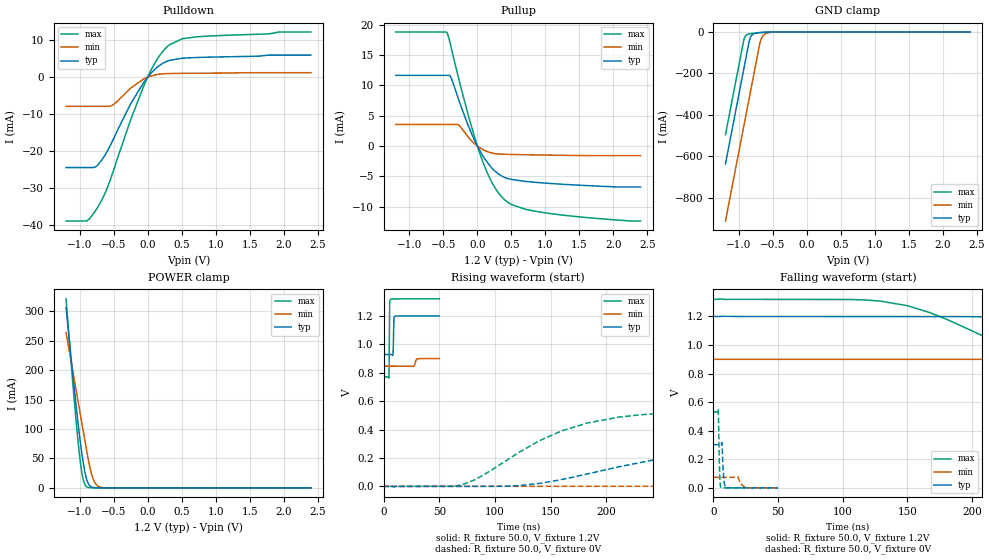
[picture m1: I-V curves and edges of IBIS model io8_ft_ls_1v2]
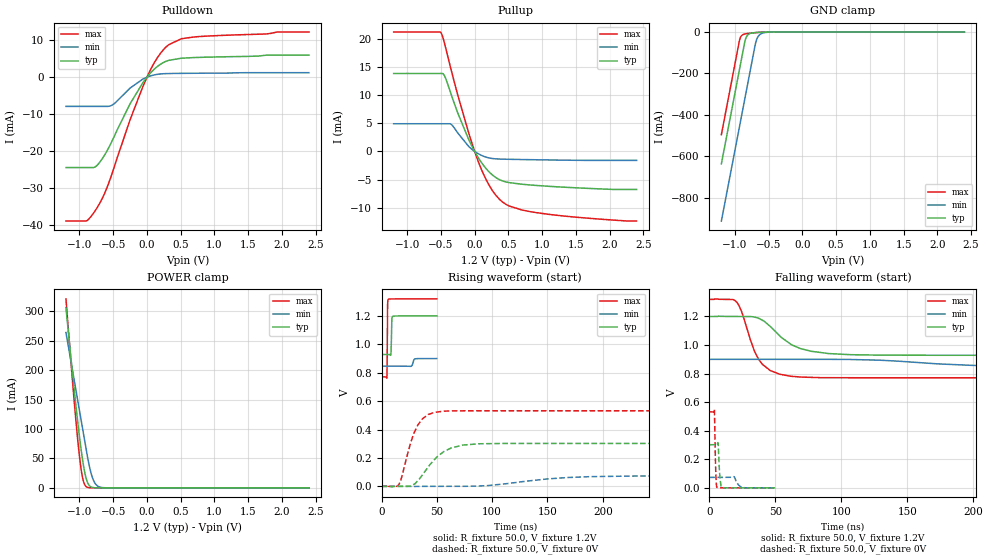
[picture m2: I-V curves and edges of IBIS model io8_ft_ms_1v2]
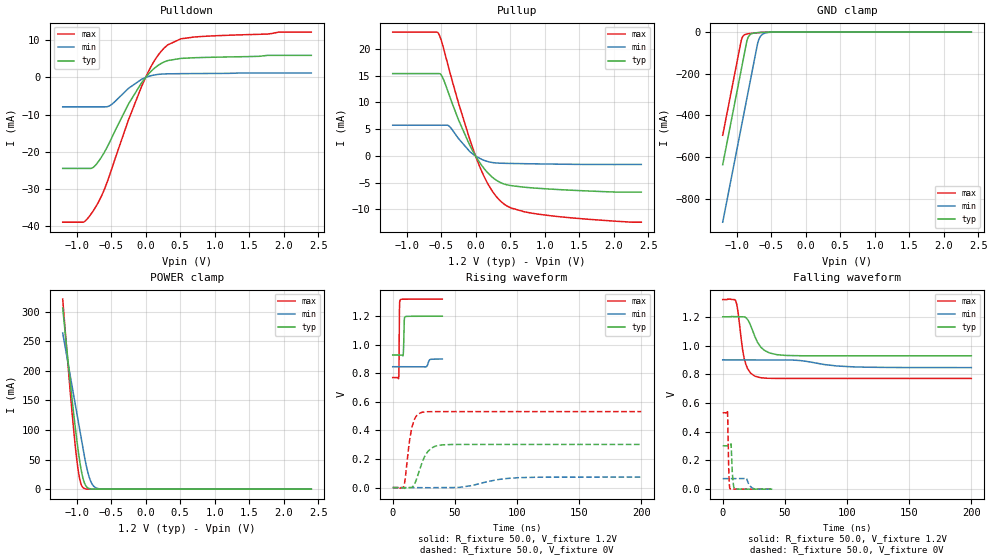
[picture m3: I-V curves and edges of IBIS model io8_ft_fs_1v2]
|   IBIS file stm32l452_lqfp64_p.ibs
[IBIS ver] 4.2
[File name] stm32l452_lqfp64_p.ibs
[File Rev] 3.0
[Date]  05-04-2021
[Source] Data Created at STMicroelectronics
[Disclaimer]  This information is for modeling purpose only and is
   not guaranted. The information is subject to change without
   notice.
[Copyright] Copyright 2021 STMicroelectronics Inc.
|   Component stm32l452_lqfp64_p
[Component] stm32l452_lqfp64_p
[Manufacturer] STMicroelectronics
[Package]
| variable   typ   min   max
R_pkg   0.0   0.0   0.0
L_pkg   0.0H   0.0H   0.0H
C_pkg   0.0F   0.0F   0.0F
[Pin]  signal_name   model_name   R_pin   L_pin   C_pin
1 VBAT POWER 68.980E-3 4.220E-9 120.000E-15
2 PC13 io8_ft 63.756E-3 3.679E-9 93.469E-15
3 PC14-OSC32_IN io8_ft 59.336E-3 3.221E-9 71.020E-15
4 PC15-OSC32_OUT io8_ft 55.719E-3 2.846E-9 52.653E-15
5 PH0-OSC_IN io8_ft 52.907E-3 2.555E-9 38.367E-15
6 PH1-OSC_OUT io8_ft 50.897E-3 2.347E-9 28.163E-15
7 NRST ioreset_ft_v33 49.692E-3 2.222E-9 22.041E-15
8 PC0 io8_ft_i2c 49.290E-3 2.180E-9 20.000E-15
9 PC1 io8_ft_i2c 49.290E-3 2.180E-9 20.000E-15
10 PC2 io8_ft 49.692E-3 2.222E-9 22.041E-15
11 PC3 io8_ft 50.897E-3 2.347E-9 28.163E-15
12 VSSA/VREF- GND 52.907E-3 2.555E-9 38.367E-15
13 VDDA/VREF+ POWER 55.719E-3 2.846E-9 52.653E-15
14 PA0 io8_ft 59.336E-3 3.221E-9 71.020E-15
15 PA1 io8_ft 63.756E-3 3.679E-9 93.469E-15
16 PA2 io8_ft 68.980E-3 4.220E-9 120.000E-15
17 PA3 io8_ft 68.980E-3 4.220E-9 120.000E-15
18 VSS GND 63.756E-3 3.679E-9 93.469E-15
19 VDD POWER 59.336E-3 3.221E-9 71.020E-15
20 PA4 io8_ft 55.719E-3 2.846E-9 52.653E-15
21 PA5 io8_ft 52.907E-3 2.555E-9 38.367E-15
22 PA6 io8_ft 50.897E-3 2.347E-9 28.163E-15
23 PA7 io8_ft_i2c 49.692E-3 2.222E-9 22.041E-15
24 PC4 io8_ft 49.290E-3 2.180E-9 20.000E-15
25 PB0 io8_ft 49.290E-3 2.180E-9 20.000E-15
26 PB1 io8_ft 49.692E-3 2.222E-9 22.041E-15
27 PB2 io8_ft 50.897E-3 2.347E-9 28.163E-15
28 PB10 io8_ft_i2c 52.907E-3 2.555E-9 38.367E-15
29 PB11 io8_ft_i2c 55.719E-3 2.846E-9 52.653E-15
30 VDD12 POWER 59.336E-3 3.221E-9 71.020E-15
31 VSS GND 63.756E-3 3.679E-9 93.469E-15
32 VDD POWER 68.980E-3 4.220E-9 120.000E-15
33 PB12 io8_ft 68.980E-3 4.220E-9 120.000E-15
34 PB13 io8_ft_i2c 63.756E-3 3.679E-9 93.469E-15
35 PB14 io8_ft_i2c 59.336E-3 3.221E-9 71.020E-15
36 PB15 io8_ft 55.719E-3 2.846E-9 52.653E-15
37 PC6 io8_ft 52.907E-3 2.555E-9 38.367E-15
38 PC7 io8_ft 50.897E-3 2.347E-9 28.163E-15
39 PC8 io8_ft 49.692E-3 2.222E-9 22.041E-15
40 PC9 io8_ft 49.290E-3 2.180E-9 20.000E-15
41 PA8 io8_ft 49.290E-3 2.180E-9 20.000E-15
42 PA9 io8_ft_i2c 49.692E-3 2.222E-9 22.041E-15
43 PA10 io8_ft_i2c 50.897E-3 2.347E-9 28.163E-15
44 PA11 io8_usb_lsfs_bcd_otg20_ft 52.907E-3 2.555E-9 38.367E-15
45 PA12 io8_usb_lsfs_bcd_otg20_ft 55.719E-3 2.846E-9 52.653E-15
46 PA13 io8_ft 59.336E-3 3.221E-9 71.020E-15
47 VSS GND 63.756E-3 3.679E-9 93.469E-15
48 VDDUSB POWER 68.980E-3 4.220E-9 120.000E-15
49 PA14 io8_ft 68.980E-3 4.220E-9 120.000E-15
50 PA15 io8_ft 63.756E-3 3.679E-9 93.469E-15
51 PC10 io8_ft 59.336E-3 3.221E-9 71.020E-15
52 PC11 io8_ft 55.719E-3 2.846E-9 52.653E-15
53 PC12 io8_ft 52.907E-3 2.555E-9 38.367E-15
54 PB3 io8_ft 50.897E-3 2.347E-9 28.163E-15
55 PB4 io8_ft_i2c 49.692E-3 2.222E-9 22.041E-15
56 PB5 io8_ft 49.290E-3 2.180E-9 20.000E-15
57 PB6 io8_ft_i2c 49.290E-3 2.180E-9 20.000E-15
58 PB7 io8_ft_i2c 49.692E-3 2.222E-9 22.041E-15
59 PH3-BOOT0 io8_ft 50.897E-3 2.347E-9 28.163E-15
60 PB8 io8_ft_i2c 52.907E-3 2.555E-9 38.367E-15
61 PB9 io8_ft_i2c 55.719E-3 2.846E-9 52.653E-15
62 VDD12 POWER 59.336E-3 3.221E-9 71.020E-15
63 VSS GND 63.756E-3 3.679E-9 93.469E-15
64 VDD POWER 68.980E-3 4.220E-9 120.000E-15
[Model Selector] io8_ft
io8_ft_ls_1v2   "GPIO - 5V tolerant - 1.2V range - Low speed"
io8_ft_ms_1v2   "GPIO - 5V tolerant - 1.2V range - Med speed"
io8_ft_fs_1v2   "GPIO - 5V tolerant - 1.2V range - Fast speed"
io8_ft_hs_1v2   "GPIO - 5V tolerant - 1.2V range - High speed"
io8_ft_ls_1v8   "GPIO - 5V tolerant - 1.8V range - Low speed"
io8_ft_ms_1v8   "GPIO - 5V tolerant - 1.8V range - Med speed"
io8_ft_fs_1v8   "GPIO - 5V tolerant - 1.8V range - Fast speed"
io8_ft_hs_1v8   "GPIO - 5V tolerant - 1.8V range - High speed"
io8_ft_ls_3v3   "GPIO - 5V tolerant - 3.3V range - Low speed"
io8_ft_ms_3v3   "GPIO - 5V tolerant - 3.3V range - Med speed"
io8_ft_fs_3v3   "GPIO - 5V tolerant - 3.3V range - Fast speed"
io8_ft_hs_3v3   "GPIO - 5V tolerant - 3.3V range - High speed"
[Model Selector] io8_ft_i2c
io8_ft_ls_1v2   "GPIO - 5V tolerant - 1.2V range - Low speed"
io8_ft_ms_1v2   "GPIO - 5V tolerant - 1.2V range - Med speed"
io8_ft_fs_1v2   "GPIO - 5V tolerant - 1.2V range - Fast speed"
io8_ft_hs_1v2   "GPIO - 5V tolerant - 1.2V range - High speed"
io8_ft_ls_1v8   "GPIO - 5V tolerant - 1.8V range - Low speed"
io8_ft_ms_1v8   "GPIO - 5V tolerant - 1.8V range - Med speed"
io8_ft_fs_1v8   "GPIO - 5V tolerant - 1.8V range - Fast speed"
io8_ft_hs_1v8   "GPIO - 5V tolerant - 1.8V range - High speed"
io8_ft_ls_3v3   "GPIO - 5V tolerant - 3.3V range - Low speed"
io8_ft_ms_3v3   "GPIO - 5V tolerant - 3.3V range - Med speed"
io8_ft_fs_3v3   "GPIO - 5V tolerant - 3.3V range - Fast speed"
io8_ft_hs_3v3   "GPIO - 5V tolerant - 3.3V range - High speed"
io8_ft_i2c_1v2   "GPIO - 5V tolerant - 1.2V range - Open drain"
io8_ft_i2c_1v8   "GPIO - 5V tolerant - 1.8V range - Open drain"
io8_ft_i2c_3v3   "GPIO - 5V tolerant - 3.3V range - Open drain"
[Model Selector] io8_usb_lsfs_bcd_otg20_ft
io8_ft_ls_1v2   "GPIO - 5V tolerant - 1.2V range - Low speed"
io8_ft_ms_1v2   "GPIO - 5V tolerant - 1.2V range - Med speed"
io8_ft_fs_1v2   "GPIO - 5V tolerant - 1.2V range - Fast speed"
io8_ft_hs_1v2   "GPIO - 5V tolerant - 1.2V range - High speed"
io8_ft_ls_1v8   "GPIO - 5V tolerant - 1.8V range - Low speed"
io8_ft_ms_1v8   "GPIO - 5V tolerant - 1.8V range - Med speed"
io8_ft_fs_1v8   "GPIO - 5V tolerant - 1.8V range - Fast speed"
io8_ft_hs_1v8   "GPIO - 5V tolerant - 1.8V range - High speed"
io8_ft_ls_3v3   "GPIO - 5V tolerant - 3.3V range - Low speed"
io8_ft_ms_3v3   "GPIO - 5V tolerant - 3.3V range - Med speed"
io8_ft_fs_3v3   "GPIO - 5V tolerant - 3.3V range - Fast speed"
io8_ft_hs_3v3   "GPIO - 5V tolerant - 3.3V range - High speed"
io8usb_ft_hs_3v3   "USB full speed"
io8usb_ft_ls_3v3   "USB low speed"
|[Model Selector] ioreset_ft_v33
|ioreset_ft_v33_1v2   "Reset PAD. 5V tolerant. 1.2V range"
|ioreset_ft_v33_1v8   "Reset PAD. 5V tolerant. 1.8V range"
|ioreset_ft_v33_3v3   "Reset PAD. 5V tolerant. 3.3V range"
[Model Selector] ioreset_ft_v33
ioreset_1v2_pu  "RESET 1.2V range with PU"
ioreset_1v2  "RESET 1.2V range"
ioreset_1v8_pu  "RESET 1.8V range with PU"
ioreset_1v8  "RESET 1.8V range"
ioreset_3v3_pu  "RESET 3.3V range with PU"
ioreset_3v3  "RESET 3.3V range"
| Models and submodels in the file (23): io8_ft_ls_1v2 (I/O), io8_ft_ms_1v2 (I/O), io8_ft_fs_1v2 (I/O), io8_ft_hs_1v2 (I/O), io8_ft_ls_1v8 (I/O), io8_ft_ms_1v8 (I/O), io8_ft_fs_1v8 (I/O), io8_ft_hs_1v8 (I/O), io8_ft_ls_3v3 (I/O), io8_ft_ms_3v3 (I/O), io8_ft_fs_3v3 (I/O), io8_ft_hs_3v3 (I/O), io8_ft_i2c_1v2 (I/O_open_drain), io8_ft_i2c_1v8 (I/O_open_drain), io8_ft_i2c_3v3 (I/O_open_drain), io8usb_ft_hs_3v3 (I/O), io8usb_ft_ls_3v3 (I/O), ioreset_1v2_pu (I/O_open_drain), ioreset_1v2 (I/O_open_drain), ioreset_1v8_pu (I/O_open_drain), ioreset_1v8 (I/O_open_drain), ioreset_3v3_pu (I/O_open_drain), ioreset_3v3 (I/O_open_drain)
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[Model]   io8_ft_ls_1v2
Model_type I/O
Polarity   Non-Inverting
Enable   Active-Low
| CAP_THRESHOLD on pad IOFT is "UDTCAPC" :
| Rising=30.00f vddiom   Falling=70.00f vddiom
| C_comp min and max val. don't necessarily correlate with the min and max pvt
| but are the smallest and greatest pad capacitance found.
| var   typ   min   max
C_comp   1.83455pF  1.76050pF  1.83491pF
|C_comp_pullup   1.06365pF  1.01770pF  1.04720pF
|C_comp_pulldown   770.90000fF  742.80001fF  787.71000fF
Vinl = 270.0mV
Vinh = 924.0mV
Vmeas = 600.0mV   | Reference voltage for timing measurements
Cref  = 50.0pF   | Timing specification test load capacitance value
Rref  = 100.0MOhm   | Timing specification test load resistance value
Vref  = 600.0mV   | Timing specification test load voltage
[Model Spec]
| TIME_THRESHOLD on pin ZIV12 is "CMOS" :
| Rising=50.00f vdd   Falling=50.00f vdd
Vinl 458.70000mV 364.70000mV 499.70000mV
Vinh 728.30000mV 548.30000mV 792.30000mV
| variable   typ   min   max
[Temperature Range] 25.0 140.0 -40.0
| variable   typ   min   max
[Voltage Range] 1.2V 900.0mV 1.32V
| variable   typ   min   max
[POWER Clamp Reference] 1.2V 900.0mV 1.32V
| variable   typ   min   max
[GND Clamp Reference] 0V 0V 0V
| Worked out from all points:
|   slope of the pulldown table from 0 to 0.18 V, typ, clamps not added: 55.6 ohm
|   slope of the pullup table from 0 to 0.18 V, typ, clamps not added: 56.3 ohm
|   GND clamp passes 1 mA (typ) near -0.61 V on its own axis
|   POWER clamp passes 1 mA (typ) near -0.81 V on its own axis
|   rising waveform, R_fixture 50.0, V_fixture 1.2V: 20-80 % time 432ps typ, 1.3ns min, 278ps max; typ from 0.928 V to 1.2 V
|   falling waveform, R_fixture 50.0, V_fixture 1.2V: 20-80 % time 167ns typ, 491ns min, 99.5ns max; typ from 1.2 V to 0.928 V
|   rising waveform, R_fixture 50.0, V_fixture 0V: 20-80 % time 127ns typ, 295ns min, 78.9ns max; typ from 0 V to 0.302 V
|   falling waveform, R_fixture 50.0, V_fixture 0V: 20-80 % time 1.14ns typ, 2.98ns min, 786ps max; typ from 0.302 V to 0 V
[POWER Clamp]
-1.2V     306.2mA    263.9mA    321.2mA
-1.09V    180mA      191mA      163.4mA
-1.05V    136.9mA    164.5mA    110.9mA
-1.01V    96.55mA    138mA      64.02mA
-960mV    52.29mA    104.9mA    20.68mA
-930mV    31.08mA    85.01mA    7.282mA
-900mV    15.67mA    65.13mA    2.025mA
-850mV    3.417mA    35.2mA     196.2uA
-800mV    570.2uA    14.97mA    18.13uA
-750mV    88.98uA    4.952mA    1.667uA
-680mV    6.495uA    823.9uA    58.96nA
2.4V      0A         0A         0A
[GND Clamp]
-1.2V     -636.9mA   -913.2mA   -495.8mA
-940mV    -194.9mA   -471.2mA   -53.78mA
-920mV    -160.9mA   -437.2mA   -28.06mA
-890mV    -109.9mA   -386.2mA   -14.28mA
-850mV    -43.09mA   -318.2mA   -9.18mA
-820mV    -18.33mA   -267.2mA   -7.516mA
-780mV    -7.695mA   -199.2mA   -5.87mA
-690mV    -2.548mA   -49.42mA   -2.9mA
-660mV    -1.868mA   -24.06mA   -2.112mA
-630mV    -1.326mA   -12.18mA   -1.447mA
-430mV    -19.32uA   -177.8uA   -8.091uA
2.4V      300pA      77.2nA     208.1pA
| variable   typ   min   max
[Pullup Reference] 1.2V 900.0mV 1.32V
| variable   typ   min   max
[Pulldown Reference] 0V 0V 0V
[Pullup]
-1.2V     11.66mA    3.558mA    18.8mA
-450mV    11.66mA    3.558mA    18.75mA
-390mV    11.34mA    3.558mA    16.48mA
-280mV    7.814mA    3.503mA    11.36mA
-110mV    2.689mA    1.153mA    4.138mA
50mV      -1.039mA   -379.5uA   -1.685mA
140mV     -2.617mA   -893.8uA   -4.276mA
240mV     -3.942mA   -1.22mA    -6.527mA
430mV     -5.313mA   -1.379mA   -9.149mA
700mV     -5.836mA   -1.444mA   -10.42mA
1.08V     -6.193mA   -1.513mA   -11.17mA
2.4V      -6.768mA   -1.592mA   -12.38mA
[Pulldown]
-1.2V     -24.47mA   -7.9mA     -38.94mA
-890mV    -24.47mA   -7.9mA     -38.83mA
-720mV    -23.49mA   -7.9mA     -34.76mA
-610mV    -20.54mA   -7.9mA     -30.69mA
-510mV    -17.01mA   -7.489mA   -25.69mA
-250mV    -7.205mA   -2.955mA   -11.53mA
0V        -16fA      0A         0A
160mV     2.97mA     779.8uA    5.417mA
320mV     4.547mA    983.4uA    8.763mA
510mV     5.135mA    1.031mA    10.4mA
700mV     5.311mA    1.057mA    10.88mA
2.4V      5.965mA    1.209mA    12.22mA
[Ramp]
dV/dt_r 181.26172mV/127.09367ns 44.06031mV/295.17618ns 319.20445mV/78.91734ns
dV/dt_f 162.93173mV/166.53891ns 32.17941mV/468.67509ns 329.57818mV/99.46975ns
R_load = 50.0
| Removed startup time: 0s 0s 0s  .
| Removed end time: 49.9ns.
[Rising Waveform]
R_fixture   = 50.0
V_fixture   = 1.2V
V_fixture_min = 900.0mV
V_fixture_max = 1.32V
0s        928.4mV    846.3mV    770.7mV
4.8ns     928.5mV    846.4mV    763.2mV
5.1ns     928.5mV    846.4mV    887.9mV
5.3ns     928.5mV    846.4mV    1.143V
5.5ns     928.5mV    846.4mV    1.284V
6.1ns     928.5mV    846.4mV    1.316V
8.4ns     926.5mV    846.4mV    1.32V
9.3ns     1.171V     846.4mV    1.32V
10.1ns    1.197V     846.4mV    1.32V
49.9ns    1.2V       899.9mV    1.32V
| Removed startup time: 0s 0s 0s  .
| Removed end time: 2.9999us.
[Falling Waveform]
R_fixture   = 50.0
V_fixture   = 1.2V
V_fixture_min = 900.0mV
V_fixture_max = 1.32V
0s        1.2V       900mV      1.32V
128.4ns   1.2V       900mV      1.309V
167.6ns   1.2V       900mV      1.227V
244ns     1.189V     900mV      938.9mV
267.2ns   1.176V     900mV      887.1mV
312.7ns   1.136V     900mV      829.5mV
416.9ns   1.017V     900mV      784.2mV
527.1ns   960.2mV    899.9mV    773.6mV
789.5ns   931.6mV    897.9mV    770.8mV
3us       928.4mV    846.4mV    770.7mV
| Removed startup time: 0s 0s 0s  .
| Removed end time: 1.9999us.
[Rising Waveform]
R_fixture   = 50.0
V_fixture   = 0V
V_fixture_min = 0V
V_fixture_max = 0V
0s        -21.55uV   -19.21uV   -16.72uV
70.8ns    -14.52uV   -5.362uV   12.13mV
121.2ns   5.11mV     -2.911uV   237.5mV
159.7ns   48.13mV    4.858uV    390.3mV
210.7ns   136.7mV    43.95uV    487mV
277.5ns   227.6mV    269.3uV    522.7mV
328.2ns   266.1mV    1.529mV    529.1mV
483.4ns   299.5mV    19.45mV    532mV
966.6ns   302.1mV    70.44mV    532mV
2us       302.1mV    73.43mV    532mV
| Removed startup time: 0s 0s 0s  .
| Removed end time: 49.9ns.
[Falling Waveform]
R_fixture   = 50.0
V_fixture   = 0V
V_fixture_min = 0V
V_fixture_max = 0V
0s        302.1mV    73.45mV    532mV
3.9ns     302.1mV    73.44mV    547.9mV
4.8ns     302mV      73.44mV    150.4mV
5.8ns     301.1mV    73.44mV    2.967mV
6.7ns     315mV      73.44mV    1.089mV
8.1ns     72.96mV    73.44mV    240.9uV
9.7ns     1.263mV    73.44mV    103.6uV
18.9ns    18.32uV    77.83mV    27.76uV
26.1ns    15.27uV    960.1uV    26.42uV
49.9ns    16.04uV    8.939uV    27.43uV
[Model]   io8_ft_ms_1v2
Model_type I/O
Polarity   Non-Inverting
Enable   Active-Low
| CAP_THRESHOLD on pad IOFT is "UDTCAPC" :
| Rising=30.00f vddiom   Falling=70.00f vddiom
| C_comp min and max val. don't necessarily correlate with the min and max pvt
| but are the smallest and greatest pad capacitance found.
| var   typ   min   max
C_comp   1.83454pF  1.76050pF  1.83490pF
|C_comp_pullup   1.06365pF  1.01770pF  1.04720pF
|C_comp_pulldown   770.89000fF  742.80001fF  787.70000fF
Vinl = 270.0mV
Vinh = 924.0mV
Vmeas = 600.0mV   | Reference voltage for timing measurements
Cref  = 50.0pF   | Timing specification test load capacitance value
Rref  = 100.0MOhm   | Timing specification test load resistance value
Vref  = 600.0mV   | Timing specification test load voltage
[Model Spec]
| TIME_THRESHOLD on pin ZIV12 is "CMOS" :
| Rising=50.00f vdd   Falling=50.00f vdd
Vinl 458.70000mV 364.70000mV 499.70000mV
Vinh 728.30000mV 548.30000mV 792.30000mV
| variable   typ   min   max
[Temperature Range] 25.0 140.0 -40.0
| variable   typ   min   max
[Voltage Range] 1.2V 900.0mV 1.32V
| variable   typ   min   max
[POWER Clamp Reference] 1.2V 900.0mV 1.32V
| variable   typ   min   max
[GND Clamp Reference] 0V 0V 0V
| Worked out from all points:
|   slope of the pulldown table from 0 to 0.18 V, typ, clamps not added: 55.6 ohm
|   slope of the pullup table from 0 to 0.18 V, typ, clamps not added: 56.3 ohm
|   GND clamp passes 1 mA (typ) near -0.61 V on its own axis
|   POWER clamp passes 1 mA (typ) near -0.81 V on its own axis
|   rising waveform, R_fixture 50.0, V_fixture 1.2V: 20-80 % time 434ps typ, 1.31ns min, 279ps max; typ from 0.928 V to 1.2 V
|   falling waveform, R_fixture 50.0, V_fixture 1.2V: 20-80 % time 22.8ns typ, 62.2ns min, 13.6ns max; typ from 1.2 V to 0.928 V
|   rising waveform, R_fixture 50.0, V_fixture 0V: 20-80 % time 20.6ns typ, 53.2ns min, 12.7ns max; typ from 0 V to 0.302 V
|   falling waveform, R_fixture 50.0, V_fixture 0V: 20-80 % time 1.14ns typ, 2.98ns min, 785ps max; typ from 0.302 V to 0 V
[POWER Clamp]
-1.2V     306.2mA    263.9mA    321.2mA
-1.09V    180mA      191mA      163.4mA
-1.05V    136.9mA    164.5mA    110.9mA
-1.01V    96.55mA    138mA      64.02mA
-960mV    52.29mA    104.9mA    20.68mA
-930mV    31.08mA    85.01mA    7.282mA
-900mV    15.67mA    65.13mA    2.025mA
-850mV    3.417mA    35.2mA     196.2uA
-800mV    570.2uA    14.97mA    18.13uA
-750mV    88.98uA    4.952mA    1.667uA
-680mV    6.495uA    823.9uA    58.96nA
2.4V      0A         0A         0A
[GND Clamp]
-1.2V     -636.9mA   -913.2mA   -495.8mA
-940mV    -194.9mA   -471.2mA   -53.78mA
-920mV    -160.9mA   -437.2mA   -28.06mA
-890mV    -109.9mA   -386.2mA   -14.28mA
-850mV    -43.09mA   -318.2mA   -9.18mA
-820mV    -18.33mA   -267.2mA   -7.516mA
-780mV    -7.695mA   -199.2mA   -5.87mA
-690mV    -2.548mA   -49.42mA   -2.9mA
-660mV    -1.868mA   -24.06mA   -2.112mA
-630mV    -1.326mA   -12.18mA   -1.447mA
-430mV    -19.32uA   -177.8uA   -8.091uA
2.4V      300pA      77.2nA     208.1pA
| variable   typ   min   max
[Pullup Reference] 1.2V 900.0mV 1.32V
| variable   typ   min   max
[Pulldown Reference] 0V 0V 0V
[Pullup]
-1.2V     13.87mA    4.927mA    21.25mA
-500mV    13.87mA    4.927mA    21.15mA
-450mV    13.53mA    4.927mA    19.38mA
-350mV    10.23mA    4.844mA    14.6mA
-90mV     2.161mA    908.5uA    3.352mA
40mV      -840.8uA   -309uA     -1.362mA
130mV     -2.46mA    -847.3uA   -4.016mA
230mV     -3.829mA   -1.199mA   -6.331mA
420mV     -5.274mA   -1.376mA   -9.06mA
510mV     -5.544mA   -1.401mA   -9.708mA
900mV     -6.043mA   -1.482mA   -10.87mA
2.4V      -6.768mA   -1.593mA   -12.38mA
[Pulldown]
-1.2V     -24.47mA   -7.9mA     -38.94mA
-890mV    -24.47mA   -7.9mA     -38.83mA
-720mV    -23.49mA   -7.9mA     -34.76mA
-610mV    -20.54mA   -7.9mA     -30.69mA
-510mV    -17.01mA   -7.49mA    -25.69mA
-250mV    -7.205mA   -2.955mA   -11.53mA
0V        -16fA      0A         0A
160mV     2.97mA     779.9uA    5.417mA
320mV     4.547mA    983.4uA    8.763mA
510mV     5.135mA    1.031mA    10.4mA
700mV     5.311mA    1.057mA    10.88mA
2.4V      5.965mA    1.209mA    12.22mA
[Ramp]
dV/dt_r 181.26477mV/20.56352ns 44.07195mV/53.14365ns 319.20364mV/12.72223ns
dV/dt_f 162.9258mV/22.80306ns 32.17064mV/62.22543ns 329.54886mV/13.59962ns
R_load = 50.0
| Removed startup time: 0s 0s 0s  .
| Removed end time: 49.9ns.
[Rising Waveform]
R_fixture   = 50.0
V_fixture   = 1.2V
V_fixture_min = 900.0mV
V_fixture_max = 1.32V
0s        928.4mV    846.3mV    770.7mV
4.8ns     928.5mV    846.4mV    763.4mV
5.1ns     928.5mV    846.4mV    885.5mV
5.3ns     928.5mV    846.4mV    1.14V
5.5ns     928.5mV    846.4mV    1.283V
6.1ns     928.5mV    846.4mV    1.316V
8.4ns     926.3mV    846.4mV    1.319V
9.3ns     1.171V     846.4mV    1.319V
10.1ns    1.197V     846.4mV    1.32V
49.9ns    1.2V       899.9mV    1.32V
| Removed startup time: 0s 0s 0s  .
| Removed end time: 399.9ns.
[Falling Waveform]
R_fixture   = 50.0
V_fixture   = 1.2V
V_fixture_min = 900.0mV
V_fixture_max = 1.32V
0s        1.2V       900mV      1.32V
20.9ns    1.2V       900.5mV    1.3V
24.4ns    1.2V       900.4mV    1.237V
37.4ns    1.188V     900.1mV    899.9mV
46.1ns    1.132V     900mV      822mV
61.1ns    1.01V      900mV      782.1mV
77.1ns    956.5mV    900mV      773.7mV
106.9ns   932.6mV    899mV      770.8mV
210.5ns   928.5mV    855.2mV    770.7mV
399.9ns   928.5mV    846.4mV    770.8mV
| Removed startup time: 0s 0s 0s  .
| Removed end time: 399.9ns.
[Rising Waveform]
R_fixture   = 50.0
V_fixture   = 0V
V_fixture_min = 0V
V_fixture_max = 0V
0s        -21.53uV   -19.2uV    -16.71uV
15.6ns    -135.7uV   13.87nV    10.31mV
26.1ns    2.219mV    28.98uV    301.7mV
32.6ns    37.63mV    -253.4uV   429.5mV
36.6ns    76.23mV    -32.36uV   472.9mV
47.3ns    183.6mV    -27.66uV   520mV
63ns      270.3mV    15.69uV    531.1mV
88ns      299.6mV    2.266mV    532mV
188.8ns   302.1mV    68.31mV    532mV
399.9ns   302.1mV    73.45mV    532mV
| Removed startup time: 0s 0s 0s  .
| Removed end time: 49.9ns.
[Falling Waveform]
R_fixture   = 50.0
V_fixture   = 0V
V_fixture_min = 0V
V_fixture_max = 0V
0s        302.1mV    73.47mV    532mV
3.9ns     302.1mV    73.45mV    546.9mV
4.8ns     302mV      73.45mV    150.2mV
5.8ns     301.2mV    73.45mV    3.196mV
6.7ns     314.3mV    73.45mV    1.275mV
7.9ns     95.79mV    73.46mV    467.5uV
9.5ns     1.819mV    73.46mV    310.4uV
18.9ns    124.6uV    77.56mV    258.3uV
25.3ns    121.1uV    2.105mV    174.8uV
49.9ns    63.52uV    25.87uV    14.61uV
[Model]   io8_ft_fs_1v2
Model_type I/O
Polarity   Non-Inverting
Enable   Active-Low
| CAP_THRESHOLD on pad IOFT is "UDTCAPC" :
| Rising=30.00f vddiom   Falling=70.00f vddiom
| C_comp min and max val. don't necessarily correlate with the min and max pvt
| but are the smallest and greatest pad capacitance found.
| var   typ   min   max
C_comp   1.83456pF  1.76047pF  1.83482pF
|C_comp_pullup   1.06365pF  1.01765pF  1.04710pF
|C_comp_pulldown   770.91000fF  742.82001fF  787.72000fF
Vinl = 270.0mV
Vinh = 924.0mV
Vmeas = 600.0mV   | Reference voltage for timing measurements
Cref  = 50.0pF   | Timing specification test load capacitance value
Rref  = 100.0MOhm   | Timing specification test load resistance value
Vref  = 600.0mV   | Timing specification test load voltage
[Model Spec]
| TIME_THRESHOLD on pin ZIV12 is "CMOS" :
| Rising=50.00f vdd   Falling=50.00f vdd
Vinl 458.70000mV 364.70000mV 499.70000mV
Vinh 728.30000mV 548.30000mV 792.30000mV
| variable   typ   min   max
[Temperature Range] 25.0 140.0 -40.0
| variable   typ   min   max
[Voltage Range] 1.2V 900.0mV 1.32V
| variable   typ   min   max
[POWER Clamp Reference] 1.2V 900.0mV 1.32V
| variable   typ   min   max
[GND Clamp Reference] 0V 0V 0V
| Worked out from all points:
|   slope of the pulldown table from 0 to 0.18 V, typ, clamps not added: 55.6 ohm
|   slope of the pullup table from 0 to 0.18 V, typ, clamps not added: 56.3 ohm
|   GND clamp passes 1 mA (typ) near -0.61 V on its own axis
|   POWER clamp passes 1 mA (typ) near -0.81 V on its own axis
|   rising waveform, R_fixture 50.0, V_fixture 1.2V: 20-80 % time 436ps typ, 1.3ns min, 278ps max; typ from 0.928 V to 1.2 V
|   falling waveform, R_fixture 50.0, V_fixture 1.2V: 20-80 % time 9.24ns typ, 24.9ns min, 5.52ns max; typ from 1.2 V to 0.928 V
|   rising waveform, R_fixture 50.0, V_fixture 0V: 20-80 % time 8.19ns typ, 23ns min, 4.92ns max; typ from 0 V to 0.302 V
|   falling waveform, R_fixture 50.0, V_fixture 0V: 20-80 % time 1.14ns typ, 2.99ns min, 785ps max; typ from 0.302 V to 0 V
[POWER Clamp]
-1.2V     306.2mA    263.9mA    321.2mA
-1.09V    180mA      191mA      163.4mA
-1.05V    136.9mA    164.5mA    110.9mA
-1.01V    96.55mA    138mA      64.02mA
-960mV    52.29mA    104.9mA    20.68mA
-930mV    31.08mA    85.01mA    7.282mA
-900mV    15.67mA    65.13mA    2.025mA
-850mV    3.417mA    35.2mA     196.2uA
-800mV    570.2uA    14.97mA    18.13uA
-750mV    88.98uA    4.952mA    1.667uA
-680mV    6.495uA    823.9uA    58.96nA
2.4V      0A         0A         0A
[GND Clamp]
-1.2V     -636.9mA   -913.2mA   -495.8mA
-940mV    -194.9mA   -471.2mA   -53.78mA
-920mV    -160.9mA   -437.2mA   -28.06mA
-890mV    -109.9mA   -386.2mA   -14.28mA
-850mV    -43.09mA   -318.2mA   -9.18mA
-820mV    -18.33mA   -267.2mA   -7.516mA
-780mV    -7.695mA   -199.2mA   -5.87mA
-690mV    -2.548mA   -49.42mA   -2.9mA
-660mV    -1.868mA   -24.06mA   -2.112mA
-630mV    -1.326mA   -12.18mA   -1.447mA
-430mV    -19.32uA   -177.8uA   -8.091uA
2.4V      300pA      77.2nA     208.1pA
| variable   typ   min   max
[Pullup Reference] 1.2V 900.0mV 1.32V
| variable   typ   min   max
[Pulldown Reference] 0V 0V 0V
[Pullup]
-1.2V     15.4mA     5.746mA    23.16mA
-540mV    15.4mA     5.746mA    22.96mA
-480mV    14.75mA    5.746mA    20.88mA
-390mV    11.69mA    5.65mA     16.52mA
-250mV    6.833mA    3.296mA    10.02mA
-90mV     2.161mA    908.6uA    3.352mA
30mV      -637.7uA   -235.8uA   -1.032mA
220mV     -3.712mA   -1.175mA   -6.128mA
410mV     -5.232mA   -1.372mA   -8.966mA
510mV     -5.544mA   -1.401mA   -9.708mA
900mV     -6.043mA   -1.482mA   -10.87mA
2.4V      -6.768mA   -1.593mA   -12.38mA
[Pulldown]
-1.2V     -24.47mA   -7.9mA     -38.94mA
-890mV    -24.47mA   -7.9mA     -38.83mA
-720mV    -23.49mA   -7.9mA     -34.76mA
-610mV    -20.54mA   -7.9mA     -30.69mA
-510mV    -17.01mA   -7.49mA    -25.69mA
-250mV    -7.205mA   -2.955mA   -11.53mA
0V        -15fA      0A         0A
160mV     2.97mA     779.9uA    5.417mA
320mV     4.547mA    983.4uA    8.763mA
510mV     5.135mA    1.031mA    10.4mA
700mV     5.311mA    1.057mA    10.88mA
2.4V      5.965mA    1.209mA    12.22mA
[Ramp]
dV/dt_r 181.26153mV/8.18713ns 44.07152mV/22.97907ns 319.20813mV/4.91517ns
dV/dt_f 162.92205mV/9.23981ns 32.18237mV/24.93707ns 329.56896mV/5.51899ns
R_load = 50.0
| Removed startup time: 0s 0s 0s  .
| Removed end time: 39.9ns.
[Rising Waveform]
R_fixture   = 50.0
V_fixture   = 1.2V
V_fixture_min = 900.0mV
V_fixture_max = 1.32V
0s        928.4mV    846.3mV    770.7mV
4.8ns     928.5mV    846.4mV    763.7mV
5.1ns     928.5mV    846.4mV    884.2mV
5.3ns     928.5mV    846.4mV    1.139V
5.5ns     928.5mV    846.4mV    1.282V
6ns       928.5mV    846.4mV    1.315V
8.4ns     926.6mV    846.4mV    1.319V
9.3ns     1.17V      846.4mV    1.319V
9.9ns     1.195V     846.4mV    1.319V
39.9ns    1.2V       899.8mV    1.32V
| Removed startup time: 0s 0s 0s  .
| Removed end time: 199.9ns.
[Falling Waveform]
R_fixture   = 50.0
V_fixture   = 1.2V
V_fixture_min = 900.0mV
V_fixture_max = 1.32V
0s        1.2V       900mV      1.32V
10.2ns    1.202V     900mV      1.316V
12.3ns    1.2V       900mV      1.235V
17.2ns    1.2V       899.9mV    913.2mV
20ns      1.181V     900.7mV    839mV
25.8ns    1.064V     900.4mV    787.2mV
33.3ns    967.8mV    900.2mV    773.7mV
43.6ns    936.4mV    900mV      770.8mV
103.4ns   928.5mV    851.8mV    770.7mV
199.9ns   928.5mV    846.4mV    770.7mV
| Removed startup time: 0s 0s 0s  .
| Removed end time: 199.9ns.
[Rising Waveform]
R_fixture   = 50.0
V_fixture   = 0V
V_fixture_min = 0V
V_fixture_max = 0V
0s        -21.54uV   -19.21uV   -16.71uV
8.9ns     -3.175mV   116.4nV    6.171mV
13.8ns    -309.2uV   111.6nV    344.4mV
15.3ns    1.353mV    38.02nV    417.6mV
18.6ns    45.62mV    -273.8nV   497.4mV
23.5ns    172.6mV    13.25uV    527.2mV
31ns      276mV      -949.2uV   531.9mV
39.7ns    299.2mV    -41.11uV   532mV
101.6ns   302.1mV    69.62mV    532mV
199.9ns   302.1mV    73.45mV    532mV
| Removed startup time: 0s 0s 0s  .
| Removed end time: 39.9ns.
[Falling Waveform]
R_fixture   = 50.0
V_fixture   = 0V
V_fixture_min = 0V
V_fixture_max = 0V
0s        302.1mV    73.47mV    532mV
3.9ns     302.1mV    73.46mV    545.2mV
4.8ns     302mV      73.46mV    149.9mV
5.7ns     301.2mV    73.46mV    4.665mV
6.7ns     313.1mV    73.46mV    1.612mV
7.9ns     95.56mV    73.46mV    813.2uV
9.5ns     1.893mV    73.46mV    702.7uV
18.9ns    336.4uV    77.18mV    91.81uV
25.4ns    142.5uV    1.948mV    17.15uV
39.9ns    20.57uV    72.84uV    2.629uV
